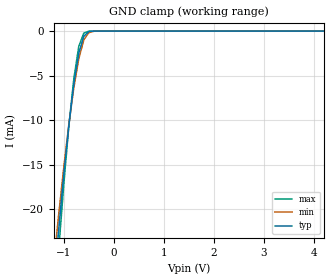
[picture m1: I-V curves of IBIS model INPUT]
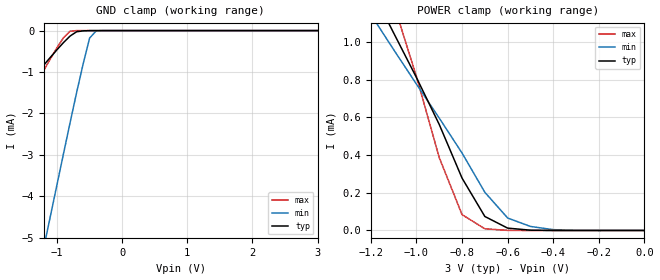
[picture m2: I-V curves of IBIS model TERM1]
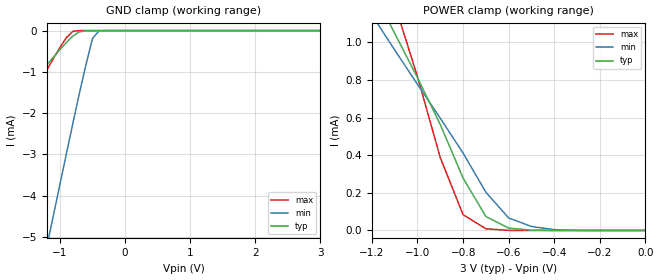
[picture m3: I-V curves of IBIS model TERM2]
|   PERICOM SEMICONDUCTOR CORP
|   IBIS Model of PI3A223
|   Product Family: 3A
|   UQFN-10 (ZM) Package
[IBIS Ver] 3.2
[Comment char] |_char
[File Name] pi3a223_zm_30v.ibs
[File Rev] 1.0
[Source] File originated at Pericom Semiconductor Corp.
[Date] 08/04/17
[Disclaimer] (C) Copyright PERICOM Semiconductor Corporation
   All rights reserved
  Pericom Semiconductor Corporation hereby grants the user of
  this IBIS model a non-exclusive, nontransferable license to
  use this IBIS model under the following terms.
  This IBIS model is provided on an "AS IS" basis and Pericom
  makes absolutely no warranty with respect to the information
  contained herein. PERICOM DISCLAIMS AND CUSTOMER WAIVES ALL
  WARRANTIES, EXPRESSED OR IMPLIED, INCLUDING WARRANTIES OF
  MERCHANTABILITY OR FITNESS FOR A PARTICULAR PURPOSE. The
  entire risk as to quality and performance is with the customer.
  Accordingly, in no event shall the company be liable for any
  damages, whether in contract or tort, including any lost
  profits or other incidental, consequential, exemplary, or
  punitive damages arising out of the use or application of the
  IBIS model provided in this package. Further, Pericom reserves
  the right to make changes without notice to any product herein
  to improve reliability, function, or design. Pericom does not
  convey any license under patent rights or any other intellectual
  property rights, including those of third parties.
  The user is granted this license only to use the IBIS model
  and is not granted rights to sell, load, rent, lease or license
  the IBIS model in whole or in part, or in modified form to anyone
  other than user. User may modify the IBIS model to suit its specific
  application but rights to derivative works and such modifications
  shall belong to Pericom.
  Pericom is not obligated to provide maintenance or support
  for the licensed IBIS model.
  Contact Pericom at ATTN: APPLICATION ENGINEERING / IBIS MODELS
  2380 Bering Drive, San Jose, CA 95131
[Component] PI3A223
[Manufacturer] Pericom Semiconductor Corp.
[Package]
| variable   typ   min   max
R_pkg   0.10120ohm   0.09060ohm   0.11180ohm
L_pkg   1.24800nH   1.01600nH   1.48000nH
C_pkg   0.22300pF   0.20300pF   0.24400pF
[Pin] signal_name   model_name   R_pin   L_pin   C_pin
1   VDD   POWER   0.10120   1.24800nH   0.22300pF
2   NO1   TERM1   0.10120   1.24800nH   0.22300pF
3   COM1   TERM2   0.11180   1.48000nH   0.24400pF
4   IN1   INPUT   0.09060   1.01600nH   0.20200pF
5   NC1   TERM1   0.11180   1.48000nH   0.24400pF
6   GND   GND   0.10120   1.24800nH   0.22300pF
7   NC2   TERM1   0.10120   1.24800nH   0.22300pF
8   IN2   INPUT   0.11180   1.48000nH   0.24400pF
9   COM2   TERM2   0.09060   1.01600nH   0.20200pF
10   NO2   TERM1   0.11180   1.48000nH   0.24400pF
[Series Switch Groups]
On 1 /
Off 2 /
[Series Pin Mapping]   pin_2   model_name  function_table_group
5   3   SWITCH1   1
2   3   SWITCH1   2
7   9   SWITCH1   1
10   9   SWITCH1   2
|   Model SWITCH1
[Model] SWITCH1
Model_type Series_switch
| variable   typ   min   max
C_comp   68.00pF   67.50pF   68.50pF
[Voltage Range]   3.0000V   2.7000V   3.3000V
[GND Clamp Reference]   0.0000V   0.0000V   0.0000V
[POWER Clamp Reference]   3.0000V   2.7000V   3.3000V
[Temperature Range]   25   85   -40
[On]
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[OFF]
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| Models and submodels in the file (4): INPUT (Input), SWITCH1 (Series_switch), TERM1 (Terminator), TERM2 (Terminator)
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|   Model INPUT
[Model] INPUT
Model_type Input
Vinl = 420mV
Vinh = 2.1V
| variable   typ   min   max
C_comp   0.950pF   0.940pF   0.960pF
[Voltage Range]   3.0000V   2.7000V   3.3000V
[GND Clamp Reference]   0.0000V   0.0000V   0.0000V
[POWER Clamp Reference]   3.0000V   2.7000V   3.3000V
[Temperature Range]   25   85   -40
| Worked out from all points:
|   GND clamp passes 1 mA (typ) near -0.62 V on its own axis
[GND Clamp]
| Voltage   I(typ)   I(min)   I(max)
-3V       -158mA     -141.6mA   -178.1mA
-1.2V     -28.62mA   -26.02mA   -32.15mA
-1.1V     -22.12mA   -20.45mA   -24.4mA
-1V       -16.06mA   -15.24mA   -17.17mA
-900mV    -10.6mA    -10.51mA   -10.7mA
-800mV    -5.96mA    -6.37mA    -5.35mA
-700mV    -2.471mA   -3.08mA    -1.693mA
-600mV    -576.6uA   -991.2uA   -224.1uA
-500mV    -63.68uA   -177.5uA   -11.66uA
-400mV    -4.071uA   -19.39uA   -283.9nA
-300mV    -171.7nA   -1.523uA   -4.445nA
6V        6.763nA    12.99nA    120.1pA
[POWER Clamp]   |Note: Vtable = Vcc - Voutput
| Voltage   I(typ)   I(min)   I(max)
-3V       0A         0A         0A
0V        0A         0A         0A
|   Model TERM1
[Model] TERM1
Model_type Terminator
| variable   typ   min   max
C_comp   27.00pF   26.70pF   27.30pF
[Voltage Range]   3.0000V   2.7000V   3.3000V
[GND Clamp Reference]   0.0000V   0.0000V   0.0000V
[POWER Clamp Reference]   3.0000V   2.7000V   3.3000V
[Temperature Range]   25   85   -40
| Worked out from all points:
|   GND clamp passes 1 mA (typ) near -1.29 V on its own axis
|   POWER clamp passes 1 mA (typ) near -1.08 V on its own axis
[GND Clamp]
| Voltage   I(typ)   I(min)   I(max)
-3V       -4.295mA   -18.87mA   -6.143mA
-2.6V     -3.516mA   -15.83mA   -4.977mA
-2.5V     -3.321mA   -15.07mA   -4.686mA
-1.2V     -826.1uA   -5.218mA   -950.2uA
-1.1V     -641.5uA   -4.465mA   -675.9uA
-900mV    -288uA     -2.968mA   -169.2uA
-800mV    -132.1uA   -2.227mA   -15.8uA
-700mV    -28.5uA    -1.5mA     -150.7nA
-600mV    -6.527uA   -810.9uA   -4.554nA
-500mV    -1.252uA   -181.6uA   -1.629nA
-400mV    -28.02nA   -7.774uA   -1.198nA
3V        322.2pA    292.4nA    251.9pA
[POWER Clamp]   |Note: Vtable = Vcc - Voutput
| Voltage   I(typ)   I(min)   I(max)
-3V       6.254mA    5.148mA    8.578mA
-1.2V     1.285mA    1.145mA    1.553mA
-1.1V     1.047mA    958.9uA    1.201mA
-1V       810.8uA    776.1uA    815.6uA
-900mV    562.1uA    596uA      386.1uA
-800mV    277.7uA    410.6uA    83.93uA
-700mV    74.19uA    202.5uA    8.974uA
-600mV    12.48uA    66.26uA    509.2nA
-500mV    1.551uA    21.36uA    15.87nA
-400mV    61.51nA    4.371uA    1.127nA
0V        318.6pA    552.7pA    347.2pA
|   Model TERM2
[Model] TERM2
Model_type Terminator
| variable   typ   min   max
C_comp   41.0pF   40.8pF   41.2pF
[Voltage Range]   3.0000V   2.7000V   3.3000V
[GND Clamp Reference]   0.0000V   0.0000V   0.0000V
[POWER Clamp Reference]   3.0000V   2.7000V   3.3000V
[Temperature Range]   25   85   -40
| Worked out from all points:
|   GND clamp passes 1 mA (typ) near -1.29 V on its own axis
|   POWER clamp passes 1 mA (typ) near -1.08 V on its own axis
[GND Clamp]
| Voltage   I(typ)   I(min)   I(max)
-3V       -4.296mA   -18.89mA   -6.144mA
-2.6V     -3.517mA   -15.85mA   -4.978mA
-2.5V     -3.322mA   -15.09mA   -4.686mA
-1.2V     -826.4uA   -5.231mA   -950.6uA
-1.1V     -641.8uA   -4.478mA   -676.2uA
-900mV    -288.2uA   -2.98mA    -169.3uA
-800mV    -132.2uA   -2.239mA   -15.8uA
-700mV    -28.52uA   -1.513mA   -150.7nA
-600mV    -6.529uA   -824.9uA   -4.556nA
-500mV    -1.253uA   -192.5uA   -1.629nA
-400mV    -28.03nA   -7.919uA   -1.196nA
3V        514.2pA    292.5nA    433.6pA
[POWER Clamp]   |Note: Vtable = Vcc - Voutput
| Voltage   I(typ)   I(min)   I(max)
-3V       6.257mA    5.15mA     8.581mA
-1.2V     1.286mA    1.146mA    1.555mA
-1.1V     1.048mA    959.5uA    1.203mA
-1V       811.9uA    776.8uA    817.4uA
-900mV    563.1uA    596.7uA    387.2uA
-800mV    278.4uA    411.4uA    84.06uA
-700mV    74.32uA    203uA      8.976uA
-600mV    12.49uA    66.4uA     509.3nA
-500mV    1.552uA    21.38uA    15.87nA
-400mV    61.54nA    4.373uA    1.155nA
0V        514.2pA    559.3pA    568.2pA
